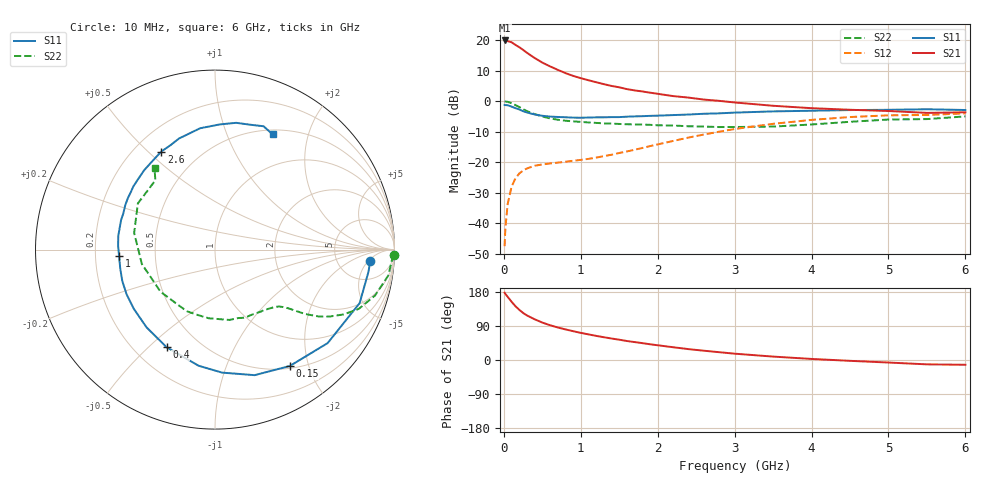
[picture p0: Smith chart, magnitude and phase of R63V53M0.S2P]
! SIEMENS Small Signal Semiconductors
! BFR193
! Si NPN RF Bipolar Junction Transistor in SOT23
! VCE = 3.5 V  IC = 3 mA
! Common Emitter S-Parameters:  May  1996
# GHz  S  MA  R  50
!  f  S11  S21  S12  S22
! GHz  MAG  ANG  MAG  ANG  MAG  ANG  MAG  ANG
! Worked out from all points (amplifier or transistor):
!   36 points, 10 MHz to 6 GHz, reference 50 ohm
!   highest |S21| = 19.9 dB at 10 MHz (marker M1)
!   |S21| within 3 dB of that: start of sweep to 245.2 MHz
!   unconditionally stable (mu >= 1): 1.041 GHz to 2.019 GHz
!   at 250 MHz: K = 0.31, MSG = 19.8 dB, |S12| = -22.7 dB
!   at 1.4 GHz: K = 1.09, MAG = 9.5 dB, |S12| = -17.6 dB
!   at 6 GHz: K = 0.98, MSG = 0.2 dB, |S12| = -4.0 dB
!   S11 on the Smith chart (normalised r, x): 10 MHz: 11, -6; 150 MHz: 0.53, -1.70; 400 MHz: 0.33, -0.57; 1 GHz: 0.30, -0.03; 2.6 GHz: 0.31, +0.55; 6 GHz: 0.56, +1.47
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0.01  0.8676 -4.2  9.915 177.5  0.0042 89.5  0.9966 -1.7
0.02  0.864 -8.2  9.841 174.4  0.0083 83.5  0.9875 -3.4
0.05  0.8593 -20.3  9.669 166.6  0.0207 79.1  0.9763 -8.5
0.1  0.8157 -39.7  9.265 153.9  0.0395 70.2  0.9277 -16.0
0.15  0.7708 -57.3  8.401 142.0  0.0541 60.9  0.8665 -22.4
0.2  0.7335 -72.5  7.688 132.6  0.0652 55.2  0.8033 -26.7
0.25  0.6865 -86.7  6.952 124.2  0.073 50.0  0.7395 -30.3
0.3  0.6536 -98.0  6.232 117.6  0.079 46.6  0.6883 -32.8
0.4  0.6072 -116.4  5.118 107.5  0.0874 42.0  0.6152 -35.6
0.5  0.5771 -131.4  4.3 98.8  0.0919 39.8  0.5609 -37.3
0.6  0.5598 -143.9  3.73 91.8  0.0954 39.7  0.5226 -38.7
0.7  0.552 -153.2  3.273 85.9  0.0984 40.0  0.4973 -40.1
0.8  0.5455 -161.2  2.894 80.8  0.1018 41.1  0.4789 -41.5
1  0.5358 -176.4  2.387 71.6  0.1091 44.9  0.4581 -44.6
1.1  0.5401 177.9  2.208 67.6  0.1134 47.2  0.4488 -46.8
1.6  0.5577 153.8  1.579 50.1  0.1501 57.2  0.4187 -58.8
2.2  0.5926 131.9  1.214 33.7  0.223 60.4  0.4001 -78.4
2.6  0.6228 118.7  1.064 24.5  0.2843 57.8  0.3842 -95.1
3.5  0.6811 97.0  0.842 9.0  0.4258 44.0  0.3838 -142.3
4.5  0.7162 80.5  0.724 -2.2  0.5503 24.9  0.4598 168.3
5.5  0.7385 68.5  0.644 -11.5  0.5952 6.5  0.5095 130.7
6  0.7176 63.4  0.658 -12.6  0.6316 1.3  0.5638 126.7
